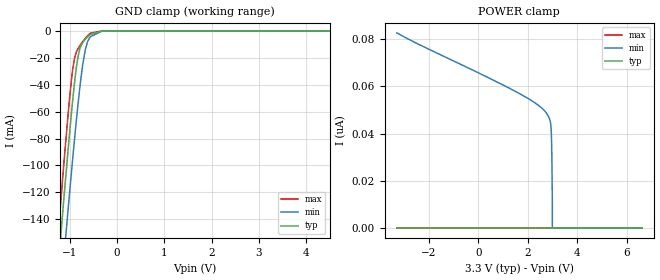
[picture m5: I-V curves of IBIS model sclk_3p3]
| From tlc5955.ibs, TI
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|   sclk_3p3 Model
[Model]   sclk_3p3
Model_type   Input
Vinl = 0.99
Vinh = 2.31
|   typ   min   max
|   (nom PVT)   (fast PVT)   (slow PVT)
C_comp   1.424e-12   1.397e-12   1.472e-12
[Model spec]
|subparameter
Vinl   0.99   0.9   1.08
Vinh   2.31   2.1   2.52
| Where nom  PVT is Nominal Process, 3.3V, 27C
|   Fast PVT is Strong Process,  3.6V, -40C
|   Slow PVT is Weak Process,   3V, 125C
[Voltage Range]   3.3   3   3.6
|Junction Temperature
[Temperature Range]   27   125   -40
[Power Clamp Reference]   3.3   3   3.6
[GND Clamp Reference]   0   0   0
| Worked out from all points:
|   GND clamp passes 1 mA (typ) near -0.42 V on its own axis
[GND Clamp]
|   Voltage   I(typ)   I(min)   I(max)
-3.3V     -1.128A    -1.136A    -1.131A
-1.3V     -198.4mA   -240.5mA   -174.2mA
-1.14V    -129.9mA   -173.9mA   -103.8mA
-1.119V   -121.2mA   -165.3mA   -94.85mA
-1.025V   -83.02mA   -127.5mA   -56.73mA
-954mV    -56.2mA    -100mA     -32.33mA
-898.8mV  -37.43mA   -79.35mA   -19.84mA
-825mV    -18.53mA   -53.42mA   -12.95mA
-675mV    -6.124mA   -14.09mA   -5.384mA
-564mV    -2.468mA   -4.147mA   -1.544mA
-246mV    -1.523uA   -28.85uA   -70.52nA
6.6V      0A         0A         0A
[POWER Clamp]
|   Voltage   I(typ)   I(min)   I(max)
-3.3V     0A         82.62nA    0A
1.605V    0A         57.27nA    0A
2.403V    0A         52.18nA    0A
2.739V    0A         48.86nA    0A
2.895V    0A         45.65nA    0A
2.943V    0A         41.92nA    0A
2.961V    0A         36.38nA    0A
2.976V    0A         26.6nA     0A
2.985V    0A         17.73nA    0A
2.991V    0A         10.45nA    0A
2.993V    0A         0A         0A
6.6V      0A         0A         0A
